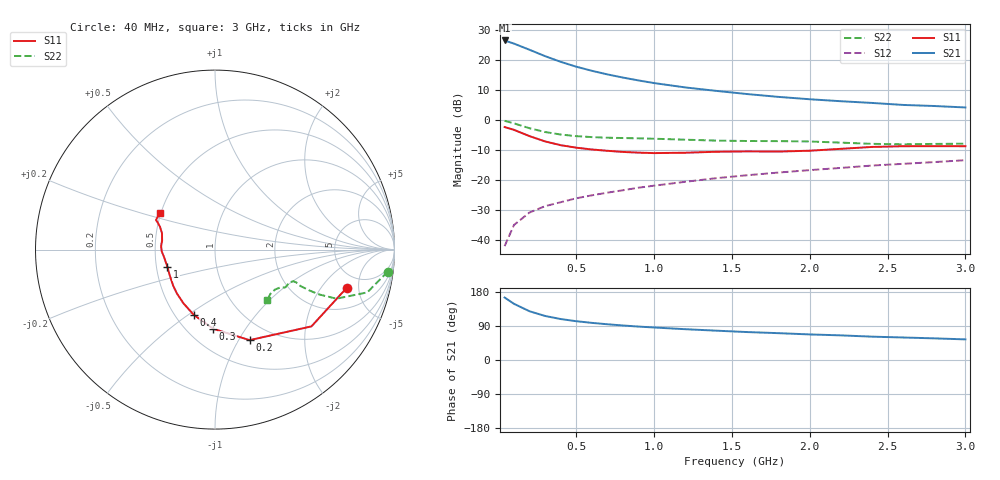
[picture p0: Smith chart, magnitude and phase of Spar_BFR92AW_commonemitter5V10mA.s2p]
! Filename:  BFR92AWC.S2P  Version:  4.0
! NXP part #: BFR92AW  Date: Jun 1994
! Bias condition: Vce=5V, Ic=10mA
#  MHz  S  MA  R  50
! Freq  S11  S21  S12  S22  !GUM [dB]
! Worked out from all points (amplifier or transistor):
!   21 points, 40 MHz to 3 GHz, reference 50 ohm
!   highest |S21| = 26.5 dB at 40 MHz (marker M1)
!   |S21| within 3 dB of that: start of sweep to 195.3 MHz
!   unconditionally stable (mu >= 1): 706.2 MHz to end of sweep
!   at 300 MHz: K = 0.68, MSG = 24.9 dB, |S12| = -28.6 dB
!   at 1 GHz: K = 1.09, MAG = 15.2 dB, |S12| = -21.8 dB
!   at 3 GHz: K = 1.08, MAG = 7.0 dB, |S12| = -13.4 dB
!   lowest NFmin = 2.00 dB at 500 MHz
!   S11 on the Smith chart (normalised r, x): 40 MHz: 3.58, -3.66; 200 MHz: 0.78, -1.11; 300 MHz: 0.66, -0.73; 400 MHz: 0.62, -0.52; 1 GHz: 0.57, -0.12; 3 GHz: 0.50, +0.23
40  0.764 -16.2  21.03 164.9  0.008 81.3  0.97 -7.3
100  0.687 -38.5  18.64 148.3  0.018 70.9  0.881 -15.7
200  0.54 -69.1  14.72 128.6  0.029 62.9  0.73 -22.0
300  0.441 -91.4  11.53 116.2  0.037 60.3  0.632 -23.3
400  0.382 -108.1  9.285 108.1  0.043 61.3  0.574 -23.4
500  0.347 -120.5  7.706 102.4  0.05 62.6  0.54 -23.2
600  0.324 -130.8  6.588 98.0  0.056 64.6  0.52 -23.1
700  0.308 -139.1  5.736 94.3  0.062 66.3  0.508 -22.9
800  0.295 -146.5  5.08 91.1  0.068 67.6  0.502 -22.6
900  0.287 -153.3  4.551 88.2  0.075 68.5  0.496 -22.3
1000  0.282 -159.8  4.118 85.8  0.081 69.5  0.489 -22.0
1200  0.286 -170.7  3.483 81.3  0.094 71.2  0.471 -22.0
1400  0.297 -178.2  3.051 77.4  0.108 72.4  0.455 -23.6
1600  0.301 176.2  2.7 73.7  0.121 72.9  0.448 -26.3
1800  0.299 170.4  2.424 70.8  0.134 74.0  0.446 -28.0
2000  0.309 162.9  2.215 67.5  0.147 74.5  0.44 -28.7
2200  0.332 157.4  2.054 65.0  0.16 74.9  0.421 -30.0
2400  0.357 154.3  1.924 61.6  0.175 75.0  0.402 -33.6
2600  0.367 153.5  1.782 59.4  0.187 75.0  0.395 -38.6
2800  0.368 151.1  1.71 57.1  0.2 75.7  0.401 -42.1
3000  0.367 146.3  1.618 54.4  0.215 75.7  0.404 -44.1
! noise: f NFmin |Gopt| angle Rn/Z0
500  2  0.293  20  0.326
1000  2.5  0.204  53.9  0.28
2000  3.4  0.199  -175.6  0.27
